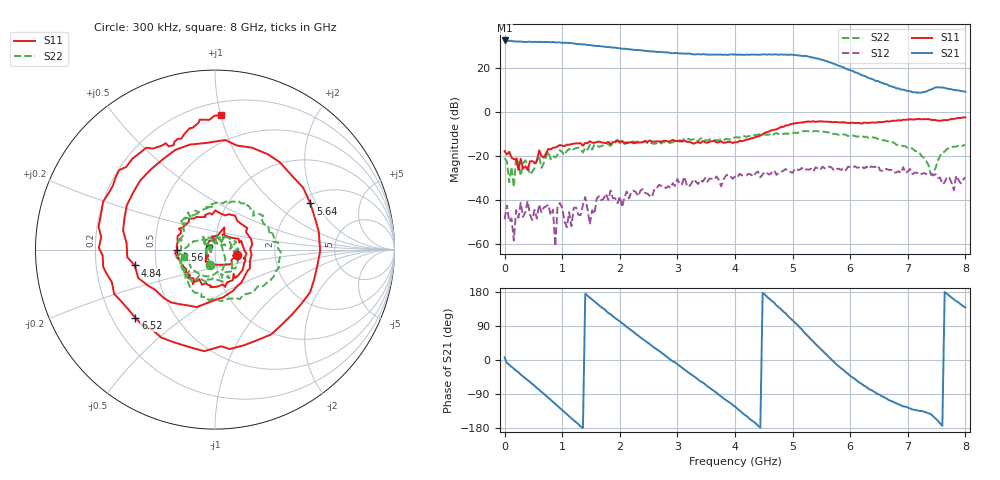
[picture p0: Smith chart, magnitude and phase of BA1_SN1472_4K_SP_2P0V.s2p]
! VC=2.00V IC=12.8mA
# HZ S DB R 50.00
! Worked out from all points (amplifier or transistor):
!   201 points, 300 kHz to 8 GHz, reference 50 ohm
!   highest |S21| = 32.3 dB at 300 kHz (marker M1)
!   |S21| within 3 dB of that: start of sweep to 1.816 GHz
!   unconditionally stable (mu >= 1): start of sweep to 2.998 GHz; 3.133 GHz to 3.66 GHz; 6.202 GHz to end of sweep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
!   at 1.32 GHz: K = 3.11, MAG = 30.9 dB, |S12| = -46.8 dB
!   at 4 GHz: K = 0.94, MSG = 27.6 dB, |S12| = -29.3 dB
!   at 8 GHz: K = 2.20, MAG = 13.2 dB, |S12| = -29.7 dB
!   S11 on the Smith chart (normalised r, x): 300 kHz: 1.28, -0.08; 2.56 GHz: 0.65, -0.01; 4.84 GHz: 0.38, -0.08; 5.64 GHz: 2.28, +1.80; 6.52 GHz: 0.30, -0.34; 8 GHz: 0.29, +1.00
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300000  -17.83 -13.1  32.32 6.9  -48.65 -115.5  -20.94 -109.1
4.02985e7  -19.31 -32.6  32.31 -7.8  -42.42 -20.7  -22.49 144.0
2.802895e8  -21.24 -128.3  31.82 -38.6  -41.19 -77.9  -29.03 -142.5
6.40276e8  -20.01 59.4  31.63 -84.4  -45.46 139.4  -25.36 44.6
8.402685e8  -16.25 18.6  31.61 -110.5  -44.34 125.1  -19.85 21.4
1.08026e9  -14.89 -19.4  31.27 -142.5  -52.28 68.4  -17.72 -16.1
1.360249e9  -15.35 -52.6  30.53 -179.3  -42.22 -53.2  -18.46 -38.2
1.680237e9  -13.85 -96.4  29.68 139.1  -40.10 -5.0  -15.55 -96.6
1.920228e9  -13.43 -123.4  29.08 110.6  -39.18 10.6  -13.93 -121.0
2.560204e9  -13.53 -178.9  27.35 37.2  -38.61 -57.5  -14.27 -178.8
2.6802e9  -13.44 172.0  27.13 24.2  -33.09 -81.9  -13.43 166.3
3.360174e9  -13.74 98.4  26.14 -51.7  -32.72 -142.9  -13.39 126.9
4.00015e9  -13.73 -7.8  25.95 -123.1  -29.30 178.2  -11.49 85.5
4.480132e9  -10.19 -101.0  26.01 177.0  -28.33 136.4  -10.30 55.1
4.840118e9  -6.83 -168.8  25.84 127.8  -26.70 98.4  -10.00 25.5
5.08011e9  -5.09 144.3  25.66 93.1  -26.13 69.6  -9.69 7.7
5.360099e9  -4.25 84.6  24.54 48.7  -26.99 59.5  -8.86 -11.0
5.640088e9  -4.58 25.8  22.48 6.1  -24.85 28.2  -9.43 -37.2
6.000075e9  -5.04 -49.1  18.82 -41.9  -24.92 -19.1  -10.89 -78.0
6.520056e9  -4.67 -139.4  13.41 -92.2  -26.53 -70.0  -12.58 -129.7
6.68005e9  -4.40 -162.5  11.77 -106.4  -26.36 -92.3  -13.47 -147.5
8e9  -2.49 87.5  9.11 138.5  -29.71 176.7  -15.14 -167.2
